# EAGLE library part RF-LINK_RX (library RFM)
RF Link receivers- WRL-8947, 8948, 8949, 8950
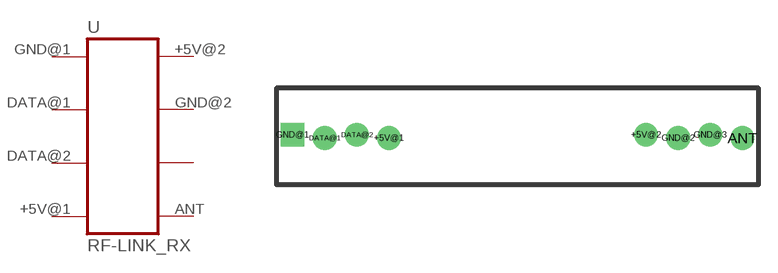
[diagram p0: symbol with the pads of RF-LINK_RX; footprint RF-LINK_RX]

Designator prefix -

## RF-LINK_RX  [RF-LINK_RX]
+5V@1  VCC1  pwr
+5V@2  VCC2  pwr
ANT  ANT
DATA@1  DATA_OUT  out
DATA@2  LINEAR_OUT  out
GND@1  GND1  pwr
GND@2  GND2  pwr
GND@3  GND3  pwr

## Footprint RF-LINK_RX (pad centres in mm)
RF-LINK receivers WRL-8947, 8948, 8949, 8950
drill 1.016 pad 1.88: +5V@1 7.62,-0.127; +5V@2 27.94,0.127; ANT 35.56,-0.127; DATA@1 2.54,-0.127; DATA@2 5.08,0.127; GND@2 30.48,-0.127; GND@3 33.02,0.127
drill 1.016 pad 1.88 square: GND@1 0,0.127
